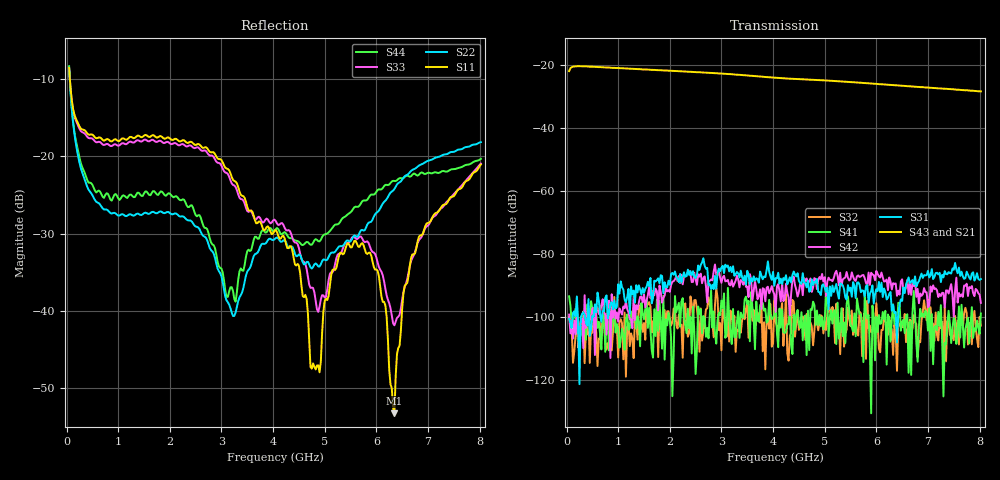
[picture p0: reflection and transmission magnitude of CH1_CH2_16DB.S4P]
!Agilent Technologies,E5071C,MY46316741,A.11.02
!Date: Thu May 28 14:27:37 2026
!Data & Calibration Information:
!1:CH1 INPUT 2:CH1 OUTPUT 3:CH2 INPUT 4:CH2 OUTPUT
!Freq	S11:SOLT4(ON)	S12:SOLT4(ON)	S13:SOLT4(ON)	S14:SOLT4(ON)
!	S21:SOLT4(ON)	S22:SOLT4(ON)	S23:SOLT4(ON)	S24:SOLT4(ON)
!	S31:SOLT4(ON)	S32:SOLT4(ON)	S33:SOLT4(ON)	S34:SOLT4(ON)
!	S41:SOLT4(ON)	S42:SOLT4(ON)	S43:SOLT4(ON)	S44:SOLT4(ON)
!PortZ  Port1:50+j0  Port2:50+j0  Port3:50+j0  Port4:50+j0
!Above PortZ is port z conversion or system Z0 setting when saving the data.
!When reading, reference impedance value at option line is always used.
# Hz S dB R 50
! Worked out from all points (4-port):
!   320 points, 50 MHz to 8.025 GHz, reference 50 ohm
!   strongest paths, dB at 50 MHz, 2.05 GHz, 4.05 GHz, 6.05 GHz, 8.025 GHz:
!     S43: -21.8, -21.7, -23.9, -25.9, -28.2
!     S21: -21.9, -21.9, -24.0, -26.0, -28.3
!     S31: -100.7, -86.0, -87.7, -88.9, -88.0
!     S42: -99.3, -88.8, -98.4, -87.1, -95.6
!     S41: -93.5, -125.3, -93.7, -99.4, -98.9
!     S32: -100.0, -101.7, -101.5, -110.1, -102.8
!   lowest |S11| = -53.3 dB at 6.35 GHz (marker M1), VSWR 1.00, Z = 50.1 + j0.156 ohm
!   |S11| at or under -10 dB: 65.13 MHz to end of sweep
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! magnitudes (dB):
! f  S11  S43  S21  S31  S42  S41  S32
! 50 MHz  -8.5  -21.8  -21.9  -100.7  -99.3  -93.5  -100.0
! 3.225 GHz  -23.0  -22.8  -22.9  -83.9  -90.4  -97.5  -104.3
! 4.75 GHz  -47.5  -24.5  -24.6  -88.1  -92.1  -97.8  -103.1
! 5.875 GHz  -32.5  -25.7  -25.8  -92.7  -89.8  -110.7  -102.8
! 6.35 GHz  -53.3  -26.3  -26.3  -98.8  -89.5  -102.3  -102.5
! 6.675 GHz  -33.1  -26.7  -26.7  -88.8  -93.0  -118.5  -101.5
! 8.025 GHz  -21.0  -28.2  -28.3  -88.0  -95.6  -98.9  -102.8
